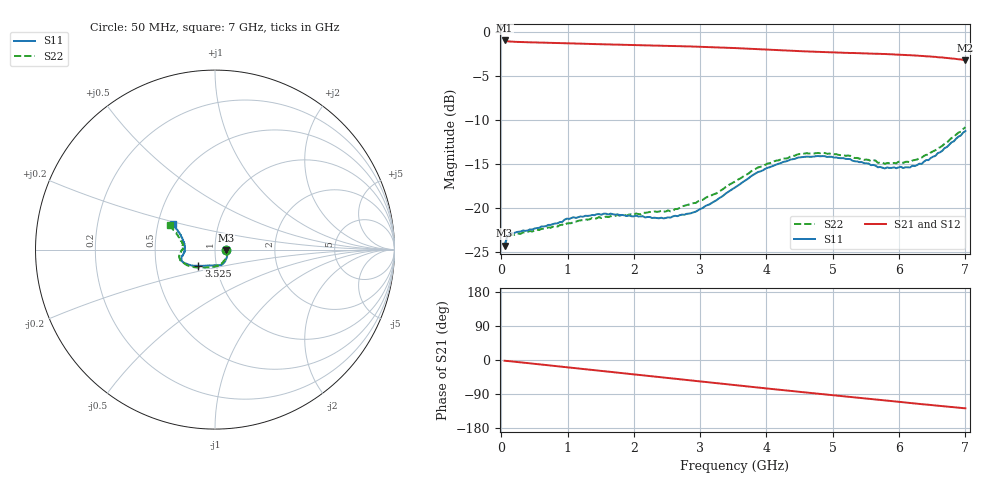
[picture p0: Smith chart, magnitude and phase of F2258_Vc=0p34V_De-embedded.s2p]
! Integrated Device Technology
! Corporate Headquarters
! 6024 Silver Creek Valley Road
! San Jose, CA 95138  USA
! Phone:  1-408-284-8200
! Toll Free:  1-800-223-1366
! Webpage:  http://www.idt.com/
! Timing and RF Division
! 515 Groton Road, Suite 102
! Westford, MA 01886-6024
! Device:  F2258
! Description: Voltage Variable RF Attenuator
! Frequency:  50.0 -  6000.00 MHz
! Package:  3x3 mm Thin QFN Plastic Package: 16 pin
! Ports:  2 RF, 2 DC
!  Pin  1  = NC
!  Pin  2  = NC
!  Pin  3  = RF2  = Port 2
!  Pin  4  = GND
!  Pin  5  = Vdd
!  Pin  6  = NC
!  Pin  7  = VCTRL
!  Pin  8  = NC
!  Pin  9  = GND
!  Pin 10  = RF1  = Port 1
!  Pin 11  = NC
!  Pin 12  = NC
!  Pin 13  = NC
!  Pin 14  = NC
!  Pin 15  = NC
!  Pin 16  = NC
! Vcntrl:  0.340 Volts
! Vdd:  +3.300 Volts
! Current:  1.089 mA
! Data:  The device was measured on a the F2258 evaluation board which has
!  individual transmission lines to the RF pins.  Data was collected
!  using a calibrated network analyzer.  The evaluation board was
!  de-embedded using a TRL calibration technique.
!  The reference plane is the edge of the package pin.
! Misc:  SN 10
!  Action Tracker AT0285
! Date Measured:  2014-12-10
! Date:  2016-01-13  MJV
! Note:
!  Integrated Device Technology supplies this data as a sample of measured
!  data at the package pin for this product.  Your particular data for this
!  product may vary.
!  Data was taken at 25 degrees C.
!  Integrated Device Technology reserves the right to change this data at anytime.
!Freq_(GHz)  S11M_(dB)  S11P_(deg)  S21M_(dB)  S21P_(deg)  S12M_(dB)  S12P_(deg)  S22M_(dB)  S22P_(deg)
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# GHz S dB R 50
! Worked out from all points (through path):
!   201 points, 50 MHz to 7 GHz, reference 50 ohm
!   highest |S21| = -0.99 dB at 50 MHz (marker M1); lowest = -3.2 dB at 7 GHz (marker M2)
!   group delay of S21, straight-line fit = 50.5 ps
!   lowest |S11| = -24.3 dB at 50 MHz (marker M3), VSWR 1.13, Z = 56.5 - j0.4 ohm
!   |S11| at or under -10 dB: start of sweep to end of sweep
!   |S22| runs from -24.4 to -10.9 dB; largest |S21 - S12| = 0.00041
!   S11 on the Smith chart (normalised r, x): 50 MHz: 1.13, -0.01; 3.525 GHz: 0.82, -0.15; 7 GHz: 0.60, +0.18
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0.05  -24.32 -3.3  -0.99 -1.9  -0.99 -1.9  -24.39 -3.1
0.08475  -23.36 -5.6  -1.07 -2.5  -1.07 -2.5  -23.48 -5.3
0.15425  -22.89 -8.8  -1.12 -3.6  -1.12 -3.6  -23.10 -9.2
0.71025  -21.97 -35.7  -1.26 -14.1  -1.26 -14.1  -22.26 -37.7
0.91875  -21.63 -45.2  -1.30 -18.0  -1.30 -18.0  -21.93 -49.2
0.98825  -21.26 -49.2  -1.31 -19.3  -1.31 -19.3  -21.80 -53.5
1.2315  -21.05 -57.4  -1.37 -23.8  -1.37 -23.8  -21.45 -62.5
1.6485  -20.69 -68.9  -1.45 -31.4  -1.45 -31.4  -20.99 -75.6
2.37825  -21.22 -89.8  -1.58 -44.8  -1.58 -44.8  -20.46 -93.4
2.552  -21.14 -95.8  -1.61 -48.0  -1.61 -48.0  -20.43 -98.6
2.93425  -20.46 -112.5  -1.69 -55.1  -1.69 -55.1  -19.47 -112.1
3.525  -17.73 -135.9  -1.86 -66.2  -1.86 -66.2  -17.05 -134.9
4.0115  -15.49 -149.9  -2.04 -75.2  -2.04 -75.2  -15.01 -150.5
4.46325  -14.34 -158.5  -2.20 -83.4  -2.20 -83.4  -13.97 -161.6
4.7065  -14.21 -161.8  -2.27 -87.7  -2.27 -87.7  -13.87 -165.9
5.2625  -14.49 -168.7  -2.42 -97.4  -2.42 -97.4  -14.11 -174.0
5.6795  -15.42 -175.4  -2.51 -104.6  -2.51 -104.6  -14.91 -179.5
5.85325  -15.49 -179.6  -2.56 -107.8  -2.56 -107.8  -14.94 175.9
6.166  -15.43 172.5  -2.67 -113.4  -2.67 -113.4  -14.86 169.9
6.33975  -15.03 166.1  -2.75 -116.5  -2.75 -116.5  -14.32 165.6
6.722  -13.11 154.2  -2.98 -123.1  -2.98 -123.1  -12.63 156.5
7  -11.29 148.6  -3.23 -127.4  -3.23 -127.4  -10.86 151.5
